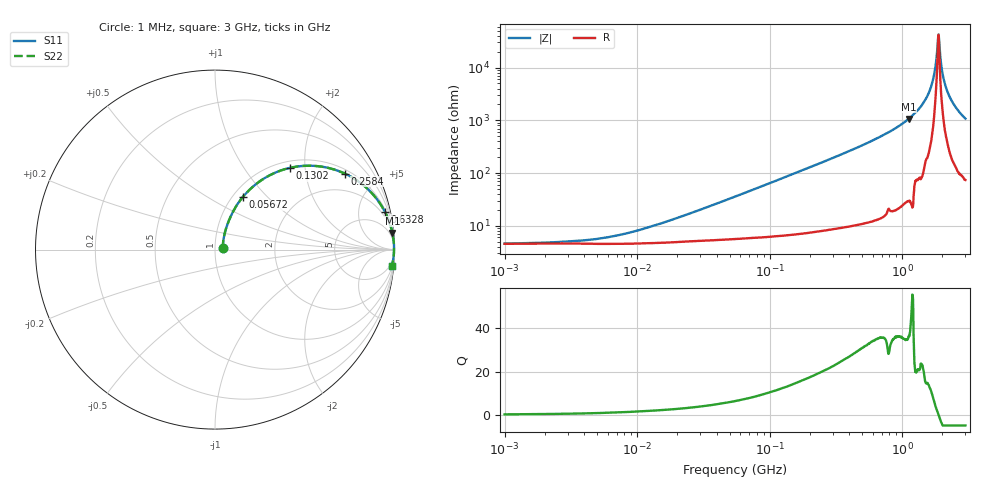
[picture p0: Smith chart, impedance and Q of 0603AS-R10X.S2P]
!s-Parameter Generated by FASTRON Sdn. Bhd.
!FASTRON P/N : 0603AS-R10X
!Keysight Technologies: E4991B_MY54100416_A.01.15
!Date created: Wed Oct 04 13:16:55 2023
!Version  : Rev01 Wed Oct 04 13:16:55 2023
!Data & Calibration Information:
!Freq	S11	S21	S12	S22
!PortZ  Port1:50+j0  Port2:50+j0
!When reading reference impedance value at option line is always used.
! Remarks : This data is being provided solely for informational purposes.
# Hz S dB R 50
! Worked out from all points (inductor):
!   1601 points, 1 MHz to 3 GHz, reference 50 ohm
!   read as one part in series: L = 104 nH near 23.05 MHz
!   highest Q = 36.4 at 1.119 GHz (marker M1), where L = 151 nH
!   self-resonance near 1.874 GHz
!   S11 on the Smith chart (normalised r, x): 1 MHz: 1.09, +0.01; 56.72 MHz: 1.11, +0.73; 130.2 MHz: 1.13, +1.66; 258.4 MHz: 1.16, +3.32; 632.8 MHz: 1.25, +8.88; 3 GHz: 2, -22
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1000000  -27.12 8.0  -0.39 -0.4  -0.39 -0.4  -27.12 8.0
3804036  -25.98 27.7  -0.39 -1.4  -0.39 -1.4  -25.98 27.7
7217957  -23.96 44.0  -0.40 -2.6  -0.40 -2.6  -23.96 44.0
1.447069e7  -19.87 58.4  -0.44 -5.2  -0.44 -5.2  -19.87 58.4
5.477226e7  -9.87 62.5  -0.93 -18.5  -0.93 -18.5  -9.87 62.5
5.672481e7  -9.61 62.1  -0.97 -19.1  -0.97 -19.1  -9.61 62.1
1.30174e8  -4.20 47.6  -2.61 -37.9  -2.61 -37.9  -4.20 47.6
2.083556e8  -2.17 35.7  -4.67 -51.1  -4.67 -51.1  -2.17 35.7
2.583764e8  -1.53 30.3  -5.93 -56.9  -5.93 -56.9  -1.53 30.3
6.327845e8  -0.27 12.6  -13.22 -75.8  -13.22 -75.8  -0.27 12.6
7.925923e8  -0.17 9.5  -15.69 -78.5  -15.69 -78.5  -0.17 9.5
1.11944e9  -0.06 5.4  -20.58 -83.1  -20.58 -83.1  -0.06 5.4
1.374365e9  -0.04 3.2  -25.04 -84.2  -25.04 -84.2  -0.04 3.2
1.589003e9  -0.02 1.7  -30.46 -84.1  -30.46 -84.1  -0.02 1.7
1.712864e9  -0.02 0.9  -35.61 -81.8  -35.61 -81.8  -0.02 0.9
1.827992e9  -0.02 0.3  -45.15 -64.8  -45.15 -64.8  -0.02 0.3
1.874306e9  -0.02 0.0  -52.45 -13.7  -52.45 -13.7  -0.02 0.0
1.931433e9  -0.02 -0.3  -45.35 64.2  -45.35 64.2  -0.02 -0.3
2.061253e9  -0.02 -1.0  -35.45 80.0  -35.45 80.0  -0.02 -1.0
2.210833e9  -0.03 -1.7  -30.54 82.5  -30.54 82.5  -0.03 -1.7
2.51802e9  -0.05 -3.1  -25.23 82.7  -25.23 82.7  -0.05 -3.1
3e9  -0.09 -5.3  -20.74 80.8  -20.74 80.8  -0.09 -5.3
